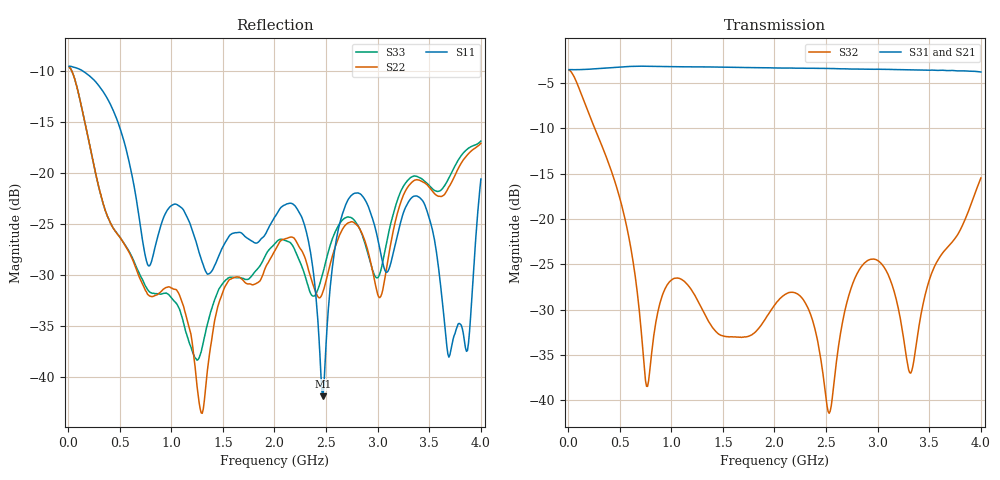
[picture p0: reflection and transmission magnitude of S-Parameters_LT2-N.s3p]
! MTS Systemtechnik GmbH
! S-Parameters
! Model: LT2-588P-4G
! Rohde & Schwarz ZVB8 2Ports - Version 3.20 - 1145.1010k08 SN: 100119
! Converted & adapted with MATLAB
!		|  MTS  |
!		|  |--o OUT 2 (Port 3)
! C (Port 1) o--| LT2-588P-4G |
!		|  |--o OUT 1 (Port 2)
! S3P File: Measurements:
! <S11,S12,S13>,
! <S21,S22,S23>,
! <S31,S32,S33>:
# HZ  S  DB  R  50.00
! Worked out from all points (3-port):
!   400 points, 10 MHz to 4 GHz, reference 50 ohm
!   strongest paths, dB at 10 MHz, 1.01 GHz, 2.01 GHz, 3.01 GHz, 4 GHz:
!     S31: -3.5, -3.2, -3.3, -3.5, -3.8
!     S21: -3.5, -3.2, -3.4, -3.5, -3.8
!     S32: -3.6, -26.7, -29.4, -24.6, -15.5
!   lowest |S11| = -41.9 dB at 2.47 GHz (marker M1), VSWR 1.02, Z = 50.6 + j0.544 ohm
!   |S11| at or under -10 dB: 135.2 MHz to end of sweep
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1e7  -9.57 177.6  -3.54 -2.7  -3.54 -2.7
     -3.54 -2.7  -9.64 171.9  -3.59 -5.5
     -3.53 -2.7  -3.59 -5.5  -9.65 171.9
3.7e8  -12.56 93.1  -3.36 -100.6  -3.35 -100.5
       -3.36 -100.6  -23.97 -51.1  -13.15 -128.4
       -3.35 -100.6  -13.16 -128.4  -23.99 -50.5
7.6e8  -28.68 -73.5  -3.16 150.3  -3.15 150.5
       -3.16 150.3  -31.71 -168.2  -38.47 -153.9
       -3.15 150.5  -38.43 -154.0  -31.29 -164.3
1.3e9  -28.79 -7.7  -3.24 -0.4  -3.23 -0.1
       -3.24 -0.4  -43.60 -149.2  -29.95 -177.2
       -3.23 -0.2  -29.94 -177.2  -37.12 -129.2
2.01e9  -24.25 -65.8  -3.36 160.6  -3.35 161.0
        -3.36 160.7  -27.55 -130.1  -29.36 176.0
        -3.35 161.0  -29.36 176.0  -26.91 -132.8
2.47e9  -41.94 42.2  -3.41 30.6  -3.40 31.1
        -3.41 30.7  -31.67 -127.0  -37.11 100.1
        -3.40 31.1  -37.08 100.0  -29.80 -110.1
2.86e9  -22.41 -144.3  -3.49 -80.3  -3.48 -79.8
        -3.49 -80.3  -26.27 -151.7  -24.99 126.6
        -3.48 -79.8  -24.98 126.5  -26.41 -143.7
3.2e9  -25.79 -124.0  -3.54 -178.1  -3.53 -177.5
       -3.54 -178.0  -23.67 -93.3  -29.85 46.7
       -3.53 -177.5  -29.86 46.8  -22.45 -93.5
3.55e9  -26.57 144.4  -3.61 80.4  -3.60 81.0
        -3.60 80.3  -22.06 -123.5  -25.25 96.2
        -3.60 80.9  -25.24 96.4  -21.75 -117.3
4e9  -20.64 64.4  -3.78 -54.6  -3.79 -53.8
     -3.79 -54.8  -17.13 -107.5  -15.46 43.4
     -3.79 -54.0  -15.47 43.4  -16.92 -104.2
